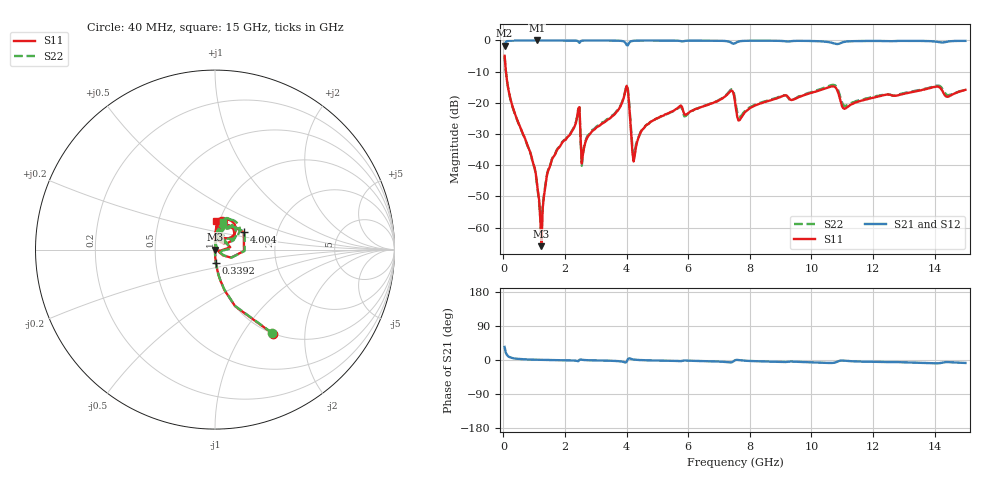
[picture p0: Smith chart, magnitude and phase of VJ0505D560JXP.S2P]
! VJ0505D560JXP
! MLCC placed on 25 mil thick microstrip substrate in series configuraton.
! DATE 06/29/2018  09:22
! CORRECTED  DATA
# GHz  S  MA  R  50.00
!  FREQ  S11M  S11A  S21M  S21A  S12M  S12A  S22M  S22A
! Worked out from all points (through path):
!   401 points, 40 MHz to 15 GHz, reference 50 ohm
!   highest |S21| = -0.01 dB at 1.087 GHz (marker M1); lowest = -1.7 dB at 40 MHz (marker M2)
!   group delay of S21, straight-line fit = 1.84 ps
!   lowest |S11| = -65.9 dB at 1.237 GHz (marker M3), VSWR 1.00, Z = 50 + j0.05 ohm
!   |S11| at or under -10 dB: 83.26 MHz to end of sweep
!   |S22| runs from -63.6 to -5.0 dB; largest |S21 - S12| = 0.0026
!   S11 on the Smith chart (normalised r, x): 40 MHz: 1.00, -1.38; 339.2 MHz: 1.00, -0.15; 4.004 GHz: 1.35, +0.27; 15 GHz: 0.96, +0.32
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0.04  0.5673 -55.6  0.8227 34.5  0.8246 34.5  0.5631 -55.5
0.3392  0.07506 -86.4  0.9955 4.3  0.9962 4.5  0.07456 -86.2
1.0872  0.005249 -91.8  0.9983 0.7  0.9985 0.8  0.005252 -88.3
1.2368  0.0005063 99.2  0.9977 0.4  0.9979 0.5  0.0006582 68.9
1.4238  0.007304 90.9  0.9975 0.1  0.9977 0.2  0.007424 87.1
1.6856  0.01522 88.9  0.9977 -0.3  0.9975 -0.2  0.01545 86.7
2.3962  0.05963 78.3  0.9835 -2.4  0.9842 -2.3  0.06079 74.7
2.5458  0.01071 35.0  0.9891 0.7  0.9894 0.7  0.00981 38.6
2.6206  0.0193 81.8  0.9946 -0.1  0.9945 -0.0  0.01998 82.4
4.0044  0.1874 31.1  0.8391 -4.8  0.8396 -4.7  0.1919 31.1
4.1914  0.01586 -13.6  0.9809 1.9  0.9811 1.9  0.01898 -10.0
4.2662  0.0146 61.2  0.9889 0.9  0.9891 0.9  0.01648 51.0
4.528  0.03793 88.5  0.9944 -0.5  0.9946 -0.4  0.03807 83.8
5.0516  0.0582 90.1  0.9949 -1.5  0.9951 -1.4  0.05784 85.0
7.3704  0.154 65.7  0.9357 -6.3  0.9366 -6.3  0.16 63.8
7.52  0.1046 27.9  0.8995 -0.7  0.9 -0.7  0.1163 26.7
7.6696  0.05283 64.4  0.9687 -0.6  0.969 -0.5  0.06008 54.9
10.0258  0.1463 83.9  0.9781 -6.2  0.9789 -6.2  0.1504 76.7
10.7364  0.1824 57.1  0.8958 -7.3  0.896 -7.3  0.1931 51.3
11.1104  0.08149 66.0  0.9558 -2.1  0.9562 -2.1  0.08925 53.4
12.5316  0.1354 81.2  0.9716 -5.6  0.972 -5.7  0.1356 72.1
15  0.1614 88.1  0.9825 -7.8  0.9832 -7.8  0.1616 74.0
